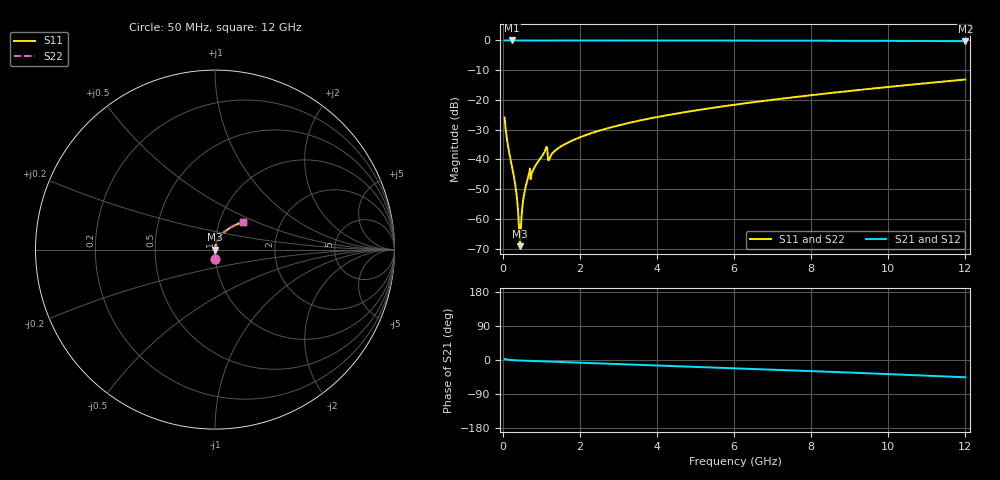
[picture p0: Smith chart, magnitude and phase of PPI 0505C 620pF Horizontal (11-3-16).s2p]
# MHz S MA R 50
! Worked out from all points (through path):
!   1601 points, 50 MHz to 12 GHz, reference 50 ohm
!   highest |S21| = 0.00 dB at 244.2 MHz (marker M1); lowest = -0.2 dB at 12 GHz (marker M2)
!   group delay of S21, straight-line fit = 10.6 ps
!   lowest |S11| = -69.2 dB at 445.8 MHz (marker M3), VSWR 1.00, Z = 50 - j0.00409 ohm
!   |S11| at or under -10 dB: start of sweep to end of sweep
!   |S22| runs from -69.2 to -13.1 dB; largest |S21 - S12| = 0
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50  0.05059 -87.0  0.9985 2.8  0.9985 2.8  0.05059 -87.0
154.5625  0.01462 -88.6  0.9996 0.4  0.9996 0.4  0.01462 -88.6
244.1875  0.007395 -88.1  0.9997 -0.3  0.9997 -0.3  0.007395 -88.1
303.9375  0.00457 -86.8  0.9997 -0.6  0.9997 -0.6  0.00457 -86.8
341.2812  0.003171 -85.1  0.9997 -0.8  0.9997 -0.8  0.003171 -85.1
408.5  0.0011 -73.4  0.9996 -1.1  0.9996 -1.1  0.0011 -73.4
445.8438  0.0003468 -6.8  0.9996 -1.3  0.9996 -1.3  0.0003468 -6.8
483.1875  0.0009721 67.1  0.9996 -1.4  0.9996 -1.4  0.0009721 67.1
535.4688  0.002159 78.5  0.9996 -1.6  0.9996 -1.6  0.002159 78.5
557.875  0.002655 80.1  0.9996 -1.7  0.9996 -1.7  0.002655 80.1
647.5  0.004654 82.5  0.9995 -2.1  0.9995 -2.1  0.004654 82.5
1088.156  0.01345 80.9  0.9986 -3.8  0.9986 -3.8  0.01345 80.9
1230.062  0.01092 78.9  0.9985 -4.1  0.9985 -4.1  0.01092 78.9
1334.625  0.01355 82.5  0.9991 -4.5  0.9991 -4.5  0.01355 82.5
1491.469  0.0162 82.8  0.9992 -5.1  0.9992 -5.1  0.0162 82.8
2044.156  0.02408 81.4  0.999 -7.2  0.999 -7.2  0.02408 81.4
2903.062  0.03587 78.7  0.9985 -10.2  0.9985 -10.2  0.03587 78.7
4038.312  0.05196 74.8  0.9976 -14.3  0.9976 -14.3  0.05196 74.8
6025  0.08321 67.7  0.9952 -21.6  0.9952 -21.6  0.08321 67.7
8019.156  0.1204 60.2  0.9911 -29.2  0.9911 -29.2  0.1204 60.2
10013.31  0.1656 52.3  0.9843 -37.2  0.9843 -37.2  0.1656 52.3
12000  0.2203 44.0  0.9732 -45.7  0.9732 -45.7  0.2203 44.0
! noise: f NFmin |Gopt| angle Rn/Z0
50  0.0003024  0.8289  0.1927  0.0003721
1372  0.003046  0.5939  3.764  0.001375
2701  0.004455  0.4899  7.117  0.001493
4031  0.005958  0.4483  10.33  0.001788
5360  0.007387  0.4214  13.39  0.002066
6682  0.00878  0.4037  16.27  0.002341
8012  0.01019  0.3927  19.02  0.00263
9341  0.01163  0.387  21.65  0.002944
1.067e+04  0.01314  0.3861  24.17  0.003295
1.2e+04  0.01474  0.3895  26.62  0.003696
